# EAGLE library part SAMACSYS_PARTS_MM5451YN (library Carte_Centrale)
MM5451YN, LED Driver, 5-Digits, 5 V, 9 V, 40-Pin PDIP Source: Datasheet
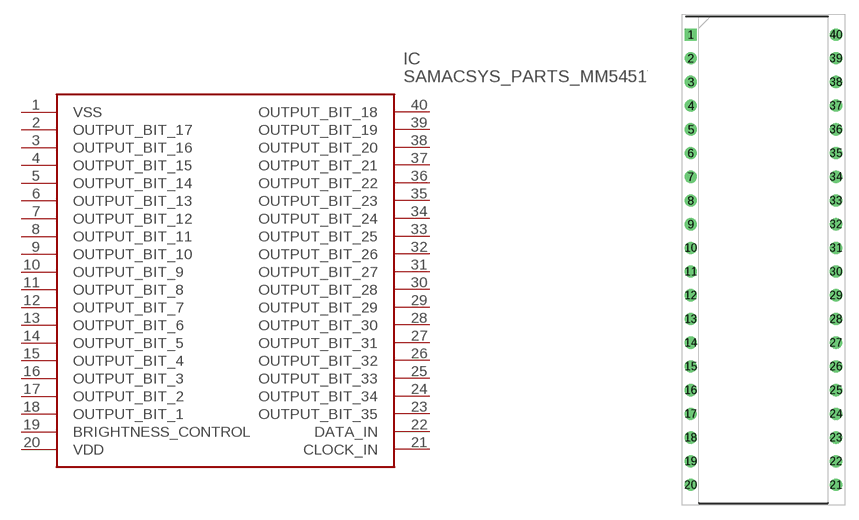
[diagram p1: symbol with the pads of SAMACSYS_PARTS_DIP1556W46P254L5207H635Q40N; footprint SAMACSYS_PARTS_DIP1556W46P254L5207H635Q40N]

Designator prefix IC

## SAMACSYS_PARTS_MM5451YN (DESCRIPTION: MM5451YN, LED Driver, 5-Digits, 5 V, 9 V, 40-Pin PDIP; HEIGHT: 6.35mm; MANUFACTURER_NAME: Micrel; MANUFACTURER_PART_NUMBER: MM5451YN; MOUSER_PART_NUMBER: 998-MM5451YN; MOUSER_PRICE-STOCK: https://www.mouser.com/Search/Refine.aspx?Keyword=998-MM5451YN)  [SAMACSYS_PARTS_DIP1556W46P254L5207H635Q40N]
1  VSS
2  OUTPUT_BIT_17
3  OUTPUT_BIT_16
4  OUTPUT_BIT_15
5  OUTPUT_BIT_14
6  OUTPUT_BIT_13
7  OUTPUT_BIT_12
8  OUTPUT_BIT_11
9  OUTPUT_BIT_10
10  OUTPUT_BIT_9
11  OUTPUT_BIT_8
12  OUTPUT_BIT_7
13  OUTPUT_BIT_6
14  OUTPUT_BIT_5
15  OUTPUT_BIT_4
16  OUTPUT_BIT_3
17  OUTPUT_BIT_2
18  OUTPUT_BIT_1
19  BRIGHTNESS_CONTROL
20  VDD
21  CLOCK_IN
22  DATA_IN
23  OUTPUT_BIT_35
24  OUTPUT_BIT_34
25  OUTPUT_BIT_33
26  OUTPUT_BIT_32
27  OUTPUT_BIT_31
28  OUTPUT_BIT_30
29  OUTPUT_BIT_29
30  OUTPUT_BIT_28
31  OUTPUT_BIT_27
32  OUTPUT_BIT_26
33  OUTPUT_BIT_25
34  OUTPUT_BIT_24
35  OUTPUT_BIT_23
36  OUTPUT_BIT_22
37  OUTPUT_BIT_21
38  OUTPUT_BIT_20
39  OUTPUT_BIT_19
40  OUTPUT_BIT_18

## Footprint SAMACSYS_PARTS_DIP1556W46P254L5207H635Q40N (pad centres in mm)
PDIP-40LD-PL-1
drill 0.8 pad 1.057 square: 1 -7.779,24.13
drill 0.8 pad 1.057: 2 -7.779,21.59; 3 -7.779,19.05; 4 -7.779,16.51; 5 -7.779,13.97; 6 -7.779,11.43; 7 -7.779,8.89; 8 -7.779,6.35; 9 -7.779,3.81; 10 -7.779,1.27; 11 -7.779,-1.27; 12 -7.779,-3.81; 13 -7.779,-6.35; 14 -7.779,-8.89; 15 -7.779,-11.43; 16 -7.779,-13.97; 17 -7.779,-16.51; 18 -7.779,-19.05; 19 -7.779,-21.59; 20 -7.779,-24.13; 21 7.779,-24.13; 22 7.779,-21.59; 23 7.779,-19.05; 24 7.779,-16.51; 25 7.779,-13.97; 26 7.779,-11.43; 27 7.779,-8.89; 28 7.779,-6.35; 29 7.779,-3.81; 30 7.779,-1.27; 31 7.779,1.27; 32 7.779,3.81; 33 7.779,6.35; 34 7.779,8.89; 35 7.779,11.43; 36 7.779,13.97; 37 7.779,16.51; 38 7.779,19.05; 39 7.779,21.59; 40 7.779,24.13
